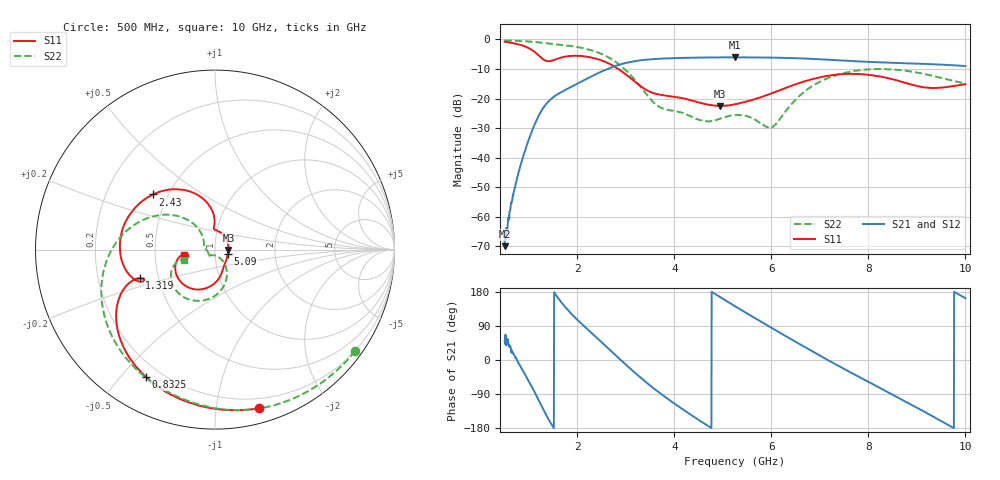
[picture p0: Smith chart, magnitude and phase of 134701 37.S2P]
!  2-Port S-parameters saved by WinCal
! VAR MeasName=S-Parameters (CALIBRATED_DATA) read from VNA (N5242A)
! VAR MeasDate=2013-7-3 16:37:13
! VAR NAME=134701 37
! VAR FILENAME=134701 37.S2P
! VAR DATE=2013-7-3 16:37:14
! VAR PHYS_PORTS=1,2
# Hz S MA R 50
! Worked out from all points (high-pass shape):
!   1601 points, 500 MHz to 10 GHz, reference 50 ohm
!   highest |S21| = -6.04 dB at 5.244 GHz (marker M1); lowest = -69.9 dB at 500 MHz (marker M2)
!   |S21| within 3 dB of the highest: 2.768 GHz to end of sweep
!   lowest |S11| = -22.5 dB at 4.947 GHz (marker M3), VSWR 1.16, Z = 58.1 - j0.32 ohm
!   |S11| at or under -10 dB: 2.847 GHz to end of sweep
!   |S22| runs from -29.9 to -0.3 dB; largest |S21 - S12| = 0.0022
!   S11 on the Smith chart (normalised r, x): 500 MHz: 0.12, -1.30; 832.5 MHz: 0.14, -0.59; 1.319 GHz: 0.39, -0.16; 2.43 GHz: 0.41, +0.32; 5.09 GHz: 1.16, -0.05; 10 GHz: 0.70, -0.04
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5e8  0.9174 -74.7  0.0003186 50.1  0.0004264 62.4  0.9632 -35.9
6.484375e8  0.8762 -94.7  0.001829 21.1  0.001785 22.2  0.954 -46.4
8.325e8  0.8075 -118.4  0.00763 -17.8  0.007647 -18.2  0.9411 -59.4
1.052188e9  0.6743 -144.7  0.02669 -68.8  0.02665 -69.1  0.9179 -75.1
1.319375e9  0.4494 -159.2  0.07387 -135.8  0.07379 -136.0  0.8732 -93.9
1.645938e9  0.4895 -161.8  0.1258 156.0  0.1255 155.8  0.8166 -115.9
2.085312e9  0.5258 165.8  0.1946 95.6  0.1937 95.5  0.723 -147.8
2.429688e9  0.4619 138.3  0.2699 55.1  0.2689 55.1  0.6007 -175.3
2.738438e9  0.3588 114.5  0.3461 18.5  0.3451 18.6  0.4468 159.5
3.047188e9  0.2392 96.4  0.4101 -17.9  0.4096 -17.8  0.2759 137.7
3.670625e9  0.1179 93.2  0.4719 -84.4  0.471 -84.4  0.07402 146.8
4.365312e9  0.09225 59.8  0.4916 -146.8  0.4918 -146.7  0.04902 -179.4
4.947188e9  0.07476 -2.1  0.4983 165.7  0.4981 165.8  0.04576 -139.9
5.089688e9  0.0764 -17.1  0.4984 154.5  0.4989 154.5  0.04983 -136.0
5.244062e9  0.08004 -31.1  0.499 142.4  0.4992 142.5  0.05253 -134.9
5.25e9  0.08 -31.7  0.4984 142.0  0.4988 142.0  0.05262 -134.8
6.01e9  0.1231 -69.6  0.4935 84.4  0.4935 84.3  0.03246 -92.2
6.835312e9  0.212 -99.7  0.4704 23.4  0.4709 23.3  0.1616 -65.9
7.494375e9  0.2599 -128.8  0.4401 -23.2  0.44 -23.4  0.2709 -94.7
8.420625e9  0.2206 -164.1  0.4059 -86.2  0.4044 -86.3  0.3142 -133.7
9.299375e9  0.1513 -167.4  0.3827 -146.8  0.3818 -146.8  0.2455 -158.7
1e10  0.1752 -170.7  0.356 163.0  0.3556 163.0  0.1811 -161.8
